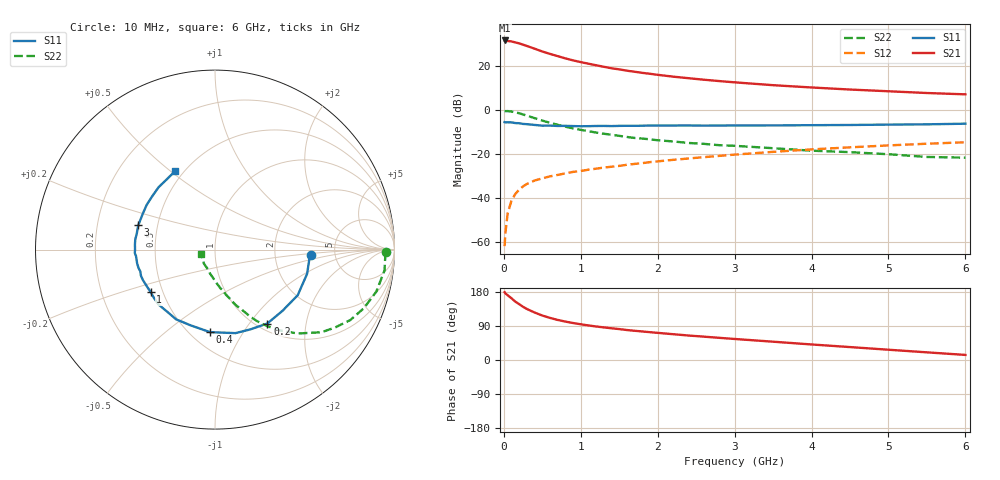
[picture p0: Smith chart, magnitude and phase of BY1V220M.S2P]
! SIEMENS Small Signal Semiconductors
! BFY420
! Si NPN RF SIEGET Grounded Emitter Transistor in MICRO-X
! VCE = 1.25 V  IC = 20 mA
! Common Emitter S-Parameters:  October  1996
# GHz  S  MA  R  50
!  f  S11  S21  S12  S22
! GHz  MAG  ANG  MAG  ANG  MAG  ANG  MAG  ANG
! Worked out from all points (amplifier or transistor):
!   36 points, 10 MHz to 6 GHz, reference 50 ohm
!   highest |S21| = 31.7 dB at 10 MHz (marker M1)
!   |S21| within 3 dB of that: start of sweep to 339 MHz
!   unconditionally stable (mu >= 1): 1.799561 GHz to 1.804726 GHz; 1.908 GHz to end of sweep
!   at 250 MHz: K = 0.31, MSG = 32.3 dB, |S12| = -34.7 dB
!   at 1.4 GHz: K = 0.93, MSG = 22.4 dB, |S12| = -25.8 dB
!   at 6 GHz: K = 1.09, MAG = 9.1 dB, |S12| = -14.6 dB
!   S11 on the Smith chart (normalised r, x): 10 MHz: 3.26, -0.30; 200 MHz: 1.11, -1.23; 400 MHz: 0.62, -0.73; 1 GHz: 0.43, -0.25; 3 GHz: 0.39, +0.13; 6 GHz: 0.45, +0.52
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0.01  0.5333 -3.5  38.62 178.8  0.0008 105.9  0.9507 -0.9
0.02  0.5281 -6.0  38.37 175.7  0.0016 93.7  0.9494 -2.3
0.05  0.5306 -14.7  37.53 170.7  0.0045 82.2  0.9517 -7.0
0.1  0.5263 -28.9  36.63 162.8  0.0088 78.5  0.9288 -14.6
0.15  0.5077 -42.1  34.86 153.9  0.0124 72.9  0.8913 -21.5
0.2  0.5046 -54.7  33.11 147.3  0.0156 69.9  0.85 -27.5
0.25  0.4861 -66.2  30.94 140.3  0.0184 65.5  0.7973 -33.0
0.3  0.4792 -76.2  28.89 134.6  0.0209 63.6  0.7512 -37.8
0.4  0.4608 -93.4  25.09 125.3  0.025 59.6  0.6565 -45.4
0.5  0.4434 -107.6  21.64 117.3  0.028 57.5  0.5783 -51.2
0.6  0.445 -119.1  19.08 111.1  0.0311 55.5  0.5158 -55.7
0.7  0.4366 -127.8  16.97 105.7  0.0335 55.3  0.4644 -59.4
0.8  0.4387 -135.6  15.1 101.4  0.0364 54.2  0.4202 -62.4
1  0.4297 -146.7  12.4 94.3  0.0412 54.5  0.3564 -66.8
1.1  0.4319 -152.7  11.42 91.2  0.0441 54.8  0.332 -69.3
1.6  0.4407 -170.2  7.915 79.1  0.0571 54.6  0.2455 -77.7
2.2  0.447 176.3  5.793 68.1  0.0739 53.1  0.194 -86.0
3  0.4483 162.4  4.298 55.5  0.0972 49.1  0.1542 -95.2
3.5  0.4492 153.8  3.703 48.3  0.1122 45.6  0.136 -101.8
4.5  0.4593 139.3  2.947 34.1  0.1424 37.1  0.1106 -114.7
5.5  0.4757 123.9  2.456 20.2  0.1721 27.6  0.086 -142.7
6  0.4915 116.6  2.291 13.4  0.1858 22.7  0.0828 -162.8
